(* Logix 5000 DataType export AMCI_NXEE2_Input_Data; software revision 20.05 *)

TYPE AMCI_NXEE2_Input_Data :
STRUCT
   Word_0_Reserved_Bit_0 : BOOL;
   Word_0_Reserved_Bit_1 : BOOL;
   CH1_Motion_Detection : BOOL;
   CH1_Velocity_at_Zero : BOOL;
   CH1_Command_Error : BOOL;
   CH1_Config_Error : BOOL;
   CH1_SSI_Setup_Error : BOOL;
   CH1_Scalar_Errors : BOOL;
   CH1_Preset_Value_Error : BOOL;
   CH1_FSC_Error : BOOL;
   CH1_FSC_Exceeded : BOOL;
   Memory_Error : BOOL;
   CH1_Input_State : BOOL;
   CH1_Value_Captured : BOOL;
   Heartbeat : BOOL;
   Acknowledge_Bit : BOOL;
   Word_1_Reserved_Bit_0 : BOOL;
   Word_1_Reserved_Bit_1 : BOOL;
   CH2_Motion_Detection : BOOL;
   CH2_Velocity_at_Zero : BOOL;
   CH2_Command_Error : BOOL;
   CH2_Config_Error : BOOL;
   CH2_SSI_Setup_Error : BOOL;
   CH2_Scalar_Errors : BOOL;
   CH2_Preset_Value_Error : BOOL;
   CH2_FSC_Error : BOOL;
   CH2_FSC_Exceeded : BOOL;
   Word_1_Reserved_bit_11 : BOOL;
   CH2_Input_State : BOOL;
   CH2_Value_Captured : BOOL;
   Word_1_Reserved_bit_14 : BOOL;
   Word_1_Reserved_bit_15 : BOOL;
   CH1_Value_1 : DINT;
   CH1_Value_2 : DINT;
   CH2_Value_1 : DINT;
   CH2_Value_2 : DINT;
END_STRUCT
END_TYPE
